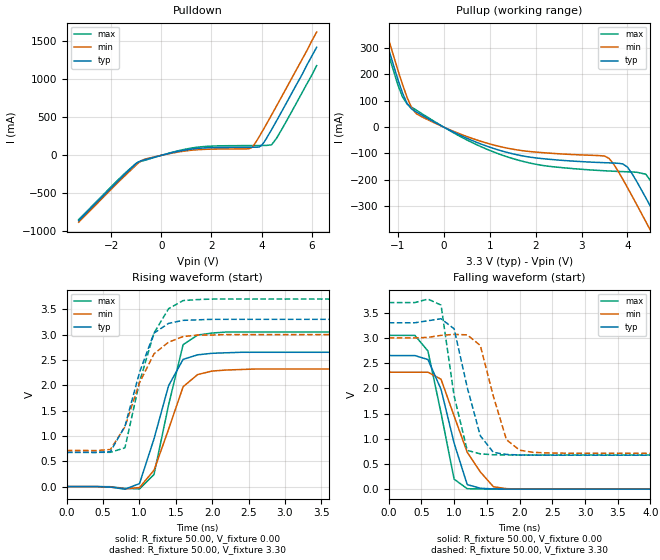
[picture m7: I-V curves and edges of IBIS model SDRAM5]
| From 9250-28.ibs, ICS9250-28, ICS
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|   Model SDRAM5
[Model]   SDRAM5
Model_type   Output
Polarity   Non-Inverting
Vmeas = 1.5V
Cref = 30pF
Rref = 0
Vref = 1.5V
C_comp   5.50pF   5.00pF   6.00pF
[Temperature Range]   27.00   70.00   0.00
[Voltage Range]   3.30V   3.00V   3.70V
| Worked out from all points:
|   slope of the pulldown table from 0 to 0.495 V, typ, clamps not added: 12.4 ohm
|   slope of the pullup table from 0 to 0.495 V, typ, clamps not added: 11.9 ohm
|   rising waveform, R_fixture 50.00, V_fixture 0.00: 20-80 % time 343ps typ, 338ps min, 285ps max; typ from 0 V to 2.65 V
|   rising waveform, R_fixture 50.00, V_fixture 3.30: 20-80 % time 333ps typ, 378ps min, 347ps max; typ from 0.674 V to 3.3 V
|   falling waveform, R_fixture 50.00, V_fixture 0.00: 20-80 % time 341ps typ, 449ps min, 288ps max; typ from 2.65 V to 0 V
|   falling waveform, R_fixture 50.00, V_fixture 3.30: 20-80 % time 301ps typ, 295ps min, 244ps max; typ from 3.3 V to 0.674 V
[Pulldown]
| voltage   I(typ)   I(min)   I(max)
-3.3V     -857.9mA   -878.4mA   -845.3mA
-1.5V     -261.3mA   -282.1mA   -248.7mA
-1V       -107.9mA   -125mA     -102.2mA
-700mV    -61.18mA   -54.61mA   -68.48mA
400mV     32.81mA    27.49mA    37.39mA
1.3V      86.08mA    70.47mA    101mA
3.6V      106.5mA    100.3mA    128.8mA
3.9V      109mA      241.5mA    129.5mA
4V        129.1mA    297.5mA    129.7mA
4.4V      337.5mA    530.4mA    138.4mA
4.8V      572.7mA    768.9mA    336.6mA
6.2V      1.42A      1.62A      1.18A
[Pullup]
| voltage   I(typ)   I(min)   I(max)
-3.3V     1.55A      1.59A      1.53A
-1.5V     466.5mA    504.3mA    443.1mA
-900mV    130.2mA    162.8mA    114.9mA
-500mV    47.62mA    41.2mA     53.65mA
1.4V      -96.88mA   -80.34mA   -113.7mA
3.5V      -134.9mA   -109.7mA   -165.5mA
4V        -151.9mA   -229.4mA   -169.5mA
4.4V      -268.3mA   -358.7mA   -178.6mA
4.6V      -333.1mA   -424.7mA   -227.1mA
4.8V      -399mA     -491.2mA   -289.4mA
5.2V      -532.3mA   -624.9mA   -420.4mA
6.2V      -869.5mA   -962.1mA   -756.3mA
[Ramp]
| variable   typ   min   max
dV/dt_r   1.59/233.66p   1.39/277.38p   1.83/212.62p
dV/dt_f   1.58/200.00p   1.37/200.00p   1.81/200.00p
[Rising Waveform]
R_fixture = 50.00
V_fixture = 0.00
V_fixture_min = 0.00
V_fixture_max = 0.00
| time   V(typ)   V(min)   V(max)
0s        0V         0V         0V
800ps     -51.3mV    -44.03mV   -35.96mV
1ns       57.46mV    -19.82mV   -46.05mV
1.2ns     943.4mV    323.6mV    239.4mV
1.4ns     1.99V      1.13V      1.61V
1.6ns     2.51V      1.97V      2.8V
1.8ns     2.6V       2.21V      2.99V
2ns       2.63V      2.28V      3.03V
2.6ns     2.65V      2.32V      3.05V
10ns      2.65V      2.32V      3.05V
[Rising Waveform]
R_fixture = 50.00
V_fixture = 3.30
V_fixture_min = 3.00
V_fixture_max = 3.70
| time   V(typ)   V(min)   V(max)
0s        673.6mV    711.3mV    675.9mV
600ps     689mV      730.8mV    676.1mV
800ps     1.19V      1.18V      764.7mV
1ns       2.25V      2.05V      2.06V
1.2ns     3.03V      2.62V      3.03V
1.4ns     3.22V      2.85V      3.51V
1.6ns     3.28V      2.96V      3.67V
1.8ns     3.29V      2.99V      3.69V
2.2ns     3.3V       3V         3.7V
10ns      3.3V       3V         3.7V
[Falling Waveform]
R_fixture = 50.00
V_fixture = 0.00
V_fixture_min = 0.00
V_fixture_max = 0.00
| time   V(typ)   V(min)   V(max)
0s        2.65V      2.32V      3.05V
400ps     2.65V      2.32V      3.05V
600ps     2.57V      2.32V      2.74V
800ps     1.98V      2.18V      1.51V
1ns       912.8mV    1.45V      198.3mV
1.2ns     90.96mV    732.3mV    9.11mV
1.4ns     18.52mV    342.4mV    3.85mV
1.6ns     4.87mV     48.45mV    1.35mV
1.8ns     1.88mV     9.85mV     456uV
10ns      0V         0V         -4.93uV
[Falling Waveform]
R_fixture = 50.00
V_fixture = 3.30
V_fixture_min = 3.00
V_fixture_max = 3.70
| time   V(typ)   V(min)   V(max)
0s        3.3V       3V         3.7V
600ps     3.34V      3.01V      3.77V
800ps     3.38V      3.05V      3.65V
1ns       3.18V      3.07V      1.85V
1.2ns     2.02V      3.06V      769.8mV
1.4ns     1.06V      2.85V      700.1mV
1.6ns     728.5mV    1.84V      682.5mV
1.8ns     689.2mV    980.4mV    678.4mV
2ns       677.3mV    773.1mV    677mV
10ns      673.6mV    711.3mV    675.9mV
